| IBIS file stm32mp251_253_255_257_tfbga361.ibs
[IBIS ver] 5.1
[File name] stm32mp251_253_255_257_tfbga361.ibs
[File Rev] 1.3
[Date] 09-10-2025
[Source] Data Created at STMicroelectronics
[Notes]  File originated from ELDO simulations.
[Disclaimer]  This information is for modeling purpose only and is
   not guaranted. The information is subject to change without
   notice.
[Copyright] Copyright 2025 STMicroelectronics Inc.
|   Component stm32mp251_253_255_257_tfbga361
[Component] stm32mp251_253_255_257_tfbga361
[Manufacturer] STMicroelectronics
[Package]
| variable   typ   min   max
R_pkg  0  NA  NA
L_pkg  0  NA  NA
C_pkg  0  NA  NA
[Pin]   signal_name   model_name
A1  VSS  gnd
A2  DSI_D3N  DPHY_IBIS
A3  DSI_D2N  DPHY_IBIS
A4  DSI_CKP  DPHY_IBIS
A5  DSI_D1N  DPHY_IBIS
A6  DSI_D0N  DPHY_IBIS
A7  VDDDSI  nc
A8  PB10  io8_tt
A9  PB0  io8_tt
A10  PB5  io8_tt_i3c
A11  PD8  io8_tt
A12  PD1  io8_tt
A13  PE0  io8_tt
A14  PE6  io8_tt
A15  PE11  io8_tt
A16  PD12  io8_tt
A17  DDR_DQ11  mal4drv27_PAD
A18  DDR_DQ9  mal4drv27_PAD
A19  VSS  gnd
B1  VDDCSI  nc
B2  DSI_D3P  DPHY_IBIS
B3  DSI_D2P  DPHY_IBIS
B4  DSI_CKN  DPHY_IBIS
B5  DSI_D1P  DPHY_IBIS
B6  DSI_D0P  DPHY_IBIS
B7  VDDA18DSI  power
B8  PB7  io8_tt
B9  PB6  io8_tt
B10  PB4  io8_tt_i3c
B11  PD0  io8_tt
B12  PD15  io8_tt_i3c
B13  PE1  io8_tt
B14  PE7  io8_tt
B15  PE9  io8_tt
B16  PB12  io8_tt
B17  DDR_DQ10  mal4drv27_PAD
B18  DDR_DQS1N  mal4drv27_PAD
B19  DDR_DQS1P  mal4drv27_PAD
C1  CSI_CKP  DPHY_IBIS_L1
C2  CSI_CKN  DPHY_IBIS_L1
C3  CSI_REXT  nc
C4  PI7  io8_tt
C5  PI6  io8_tt
C6  PG15  io8_tt
C7  DSI_REXT  nc
C8  PB1  io8_tt
C9  PB2  io8_tt
C10  PD3  io8_tt
C11  PD10  io8_tt_i3c
C12  PI10  io8_tt
C13  PE2  io8_tt
C14  PE8  io8_tt
C15  PB13  io8_tt
C16  PI11  io8_tt
C17  DDR_DQ8  mal4drv27_PAD
C18  DDR_DQ15  mal4drv27_PAD
C19  DDR_DQM1  mal4drv27_PAD
D1  CSI_D1P  DPHY_IBIS_L1
D2  CSI_D1N  DPHY_IBIS_L1
D3  VDDA18CSI  power
D4  PG8  io8_tt
D5  PI5  io8_tt
D6  PI0  io8_tt
D7  PB11  io8_tt
D8  PB8  io8_tt
D9  PD2  io8_tt
D10  PD11  io8_tt_i3c
D11  PD5  io8_tt
D12  PD14  io8_tt_i3c
D13  PE4  io8_tt
D14  PE3  io8_tt
D15  PE12  io8_tt
D16  PD13  io8_tt
D17  DDR_DQ14  mal4drv27_PAD
D18  DDR_DQ13  mal4drv27_PAD
D19  DDR_DQ12  mal4drv27_PAD
E1  CSI_D0N  DPHY_IBIS_L1
E2  CSI_D0P  DPHY_IBIS_L1
E3  PG14  io8_tt
E4  PG9  io8_tt
E5  PG10  io8_tt
E6  PG11  io8_tt
E7  PB9  io8_tt
E8  PB3  io8_tt
E9  PD9  io8_tt
E10  PD4  io8_tt
E11  PD7  io8_tt
E12  PD6  io8_tt
E13  PE5  io8_tt
E14  PE10  io8_tt
E15  PE13  io8_tt
E16  PB14  io8_tt
E17  DDR_RESETN  nc
E18  DDR_A9  mal4drv20_PAD
E19  DDR_A20  mal4drv20_PAD
F1  LVDS1_D0P  nc
F2  LVDS1_D0N  nc
F3  VDDLVDS  nc
F4  PI1  io8_tt_i3c
F5  PF14  io8_tt
F6  PG7  io8_tt
F7  VDDA18PLL3  nc
F8  VDDA18PLL2  nc
F9  VDDIO4  power
F10  VDDIO4  power
F11  VDDIO3  power
F12  VDDIO3  power
F13  VDDIO2  power
F14  VDDIO1  power
F15  PE14  io8_tt
F16  PE15  io8_tt
F17  DDR_A0  mal4drv20_PAD
F18  DDR_A11  mal4drv20_PAD
F19  DDR_A21  mal4drv20_PAD
G1  LVDS1_D1P  nc
G2  LVDS1_D1N  nc
G3  VDDA18LVDS  power
G4  PG12  io8_tt
G5  PF15  io8_tt
G6  PF13  io8_tt
G7  VSS  gnd
G8  VDDCORE  nc
G9  VSS  gnd
G10  VDDCORE  nc
G11  VSS  gnd
G12  VDDCPU  nc
G13  VSS  gnd
G14  VDDQDDR  power
G15  VSS  gnd
G16  DDR_ZQ  nc
G17  DDR_A1  mal4drv20_PAD
G18  DDR_A10  mal4drv20_PAD
G19  DDR_A22  mal4drv20_PAD
H1  LVDS1_D2P  nc
H2  LVDS1_D2N  nc
H3  PG5  io8_tt_i3c
H4  PI3  io8_tt
H5  PG13  io8_tt_i3c
H6  PI4  io8_tt
H7  VDDCORE  nc
H8  VSS  gnd
H9  VDDCORE  nc
H10  VSS  gnd
H11  VDDCPU  nc
H12  VSS  gnd
H13  VDDCPU  nc
H14  VSS  gnd
H15  VDDA18PLL1  nc
H16  VSS  gnd
H17  DDR_A25  mal4drv20_PAD
H18  DDR_A8  mal4drv20_PAD
H19  DDR_A23  mal4drv20_PAD
J1  LVDS1_D4P  nc
J2  LVDS1_D4N  nc
J3  PG6  io8_tt_i3c
J4  PI9  io8_tt
J5  PF12  io8_tt
J6  PI2  io8_tt
J7  VSS  gnd
J8  VDDCORE  nc
J9  VSS  gnd
J10  VDDCORE  nc
J11  VSS  gnd
J12  VDDCPU  nc
J13  VSS  gnd
J14  VDDQDDR  power
J15  VSS  gnd
J16  VDDA18DDR  nc
J17  DDR_A2  mal4drv20_PAD
J18  DDR_A13  mal4drv20_PAD
J19  DDR_A3  mal4drv20_PAD
K1  LVDS1_D3P  nc
K2  LVDS1_D3N  nc
K3  PZ8  io8_tt
K4  PZ6  io8_tt
K5  PC13  io8_tt
K6  V08CAP  nc
K7  VDDCORE  nc
K8  VSS  gnd
K9  VDDCORE  nc
K10  VSS  gnd
K11  VDDGPU  nc
K12  VSS  gnd
K13  VDDCPU  nc
K14  VSS  gnd
K15  VDDQDDR  power
K16  VSS  gnd
K17  DDR_VREF  nc
K18  DDR_A14  mal4drv20_PAD
K19  DDR_A26  mal4drv20_PAD
L1  PZ9  io8_tt_i3c
L2  PZ7  io8_tt
L3  PZ2  io8_tt_i3c
L4  PZ4  io8_tt_i3c
L5  PZ0  io8_tt_i3c
L6  VBAT  power
L7  VSS  gnd
L8  VDD  power
L9  VSS  gnd
L10  VDD  power
L11  VSS  gnd
L12  VDDGPU  nc
L13  VSS  gnd
L14  VDDQDDR  power
L15  VSS  gnd
L16  VDDQDDR  power
L17  DDR_A5  mal4drv20_PAD
L18  DDR_A15  mal4drv20_PAD
L19  DDR_A27  mal4drv20_PAD
M1  OSC32_OUT  isudq_tt
M2  OSC32_IN  isudq_tt
M3  PZ1  io8_tt_i3c
M4  PZ5  io8_tt
M5  PZ3  io8_tt_i3c
M6  VDDA18AON  power
M7  VSSAON  gnd
M8  VSS  gnd
M9  VDD  power
M10  VSS  gnd
M11  VDDGPU  nc
M12  VSS  gnd
M13  VDDGPU  nc
M14  VSS  gnd
M15  VDDQDDR  power
M16  VSS  gnd
M17  DDR_A4  mal4drv20_PAD
M18  DDR_A16  mal4drv20_PAD
M19  DDR_A28  mal4drv20_PAD
N1  NRST  nc
N2  PWR_CPUON  io8_tt
N3  BOOT0  isudq_tt
N4  BOOT1  isudq_tt
N5  PI8  io8_tt
N6  VDDA18ADC  power
N7  VSSA  nc
N8  VDD  power
N9  VSS  gnd
N10  VDD  power
N11  VSS  gnd
N12  VDDGPU  nc
N13  VSS  gnd
N14  VDDQDDR  power
N15  VSS  gnd
N16  VDDQDDR  power
N17  DDR_A6  mal4drv20_PAD
N18  DDR_A17  mal4drv20_PAD
N19  DDR_A29  mal4drv20_PAD
P1  PDR_ON  nc
P2  NRSTC1MS  io8_tt
P3  PWR_ON  io8_tt
P4  BOOT3  isudq_tt
P5  PA0  io8_tt
P6  PF10  io8_tt
P7  PF5  io8_tt
P8  PA14  io8_tt
P9  PA13  io8_tt
P10  PC0  io8_tt
P11  PA6  io8_tt
P12  PA7  io8_tt
P13  PH2  io8_tt_i3c
P14  PA1  io8_tt_i3c
P15  VDDPCIECLK  nc
P16  UCPD1_CC1  nc
P17  DDR_A7  mal4drv20_PAD
P18  DDR_A18  mal4drv20_PAD
P19  DDR_A30  mal4drv20_PAD
R1  OSC_IN  isudq_tt
R2  OSC_OUT  isudq_tt
R3  BOOT2  isudq_tt
R4  PF11  io8_tt
R5  PF6  io8_tt
R6  PF7  io8_tt
R7  PC5  io8_tt_i3c
R8  PA11  io8_tt
R9  PA12  io8_tt_i3c
R10  PF0  io8_tt_i3c
R11  PF2  io8_tt_i3c
R12  PH6  io8_tt_i3c
R13  PH4  io8_tt
R14  PH5  io8_tt
R15  VDDCOMBOPHYTX  nc
R16  VDD33USB  power
R17  VDDA18USB  power
R18  DDR_A12  mal4drv20_PAD
R19  DDR_A31  mal4drv20_PAD
T1  VREFN  nc
T2  VREFP  nc
T3  PG1  io8_tt_i3c
T4  PG2  io8_tt_i3c
T5  PF8  io8_tt
T6  PC4  io8_tt
T7  PC6  io8_tt_i3c
T8  PH9  io8_tt
T9  PF3  io8_tt
T10  PA2  io8_tt_i3c
T11  PA5  io8_tt
T12  PH3  io8_tt_i3c
T13  PA4  io8_tt
T14  COMBOPHY_REXT  nc
T15  VDDA18COMBOPHY  power
T16  USB3DR_TXRTUNE  nc
T17  DDR_DQM0  mal4drv27_PAD
T18  DDR_DQ5  mal4drv27_PAD
T19  DDR_DQ4  mal4drv27_PAD
U1  JTDO_TRACESWO  io8_tt
U2  NJTRST  io8_tt
U3  PG3  io8_tt
U4  PF9  io8_tt
U5  PC11  io8_tt
U6  PC7  io8_tt
U7  PC10  io8_tt
U8  PF1  io8_tt
U9  PA15  io8_tt_i3c
U10  PH7  io8_tt_i3c
U11  PH8  io8_tt
U12  PA3  io8_tt_i3c
U13  PA8  io8_tt_i3c
U14  VDDCOMBOPHY  nc
U15  UCPD1_CC2  nc
U16  USBH_HS_TXRTUNE  nc
U17  DDR_DQ3  mal4drv27_PAD
U18  DDR_DQ7  mal4drv27_PAD
U19  DDR_DQ6  mal4drv27_PAD
V1  JTCK_SWCLK  io8_tt
V2  JTMS_SWDIO  io8_tt
V3  PG4  io8_tt
V4  PC12  io8_tt_i3c
V5  PC3  io8_tt
V6  PC8  io8_tt
V7  PH12  io8_tt
V8  PC2  io8_tt
V9  PC1  io8_tt_i3c
V10  PA9  io8_tt
V11  COMBOPHY_TX1P  synopsys_usb3_tx
V12  COMBOPHY_RX1P  synopsys_usb3_rx
V13  PCIE_CLKINP  nc
V14  ANA0  nc
V15  USBH_HS_DM  USB2_HS_IBIS
V16  USB3DR_DM  USB2_HS_IBIS
V17  DDR_DQ2  mal4drv27_PAD
V18  DDR_DQS0N  mal4drv27_PAD
V19  DDR_DQS0P  mal4drv27_PAD
W1  VSS  gnd
W2  JTDI  io8_tt
W3  PB15  io8_tt
W4  PG0  io8_tt_i3c
W5  PF4  io8_tt
W6  PC9  io8_tt
W7  PH13  io8_tt
W8  PH11  io8_tt
W9  PH10  io8_tt
W10  PA10  io8_tt
W11  COMBOPHY_TX1N  synopsys_usb3_tx
W12  COMBOPHY_RX1N  synopsys_usb3_rx
W13  PCIE_CLKINN  nc
W14  ANA1  nc
W15  USBH_HS_DP  USB2_HS_IBIS
W16  USB3DR_DP  USB2_HS_IBIS
W17  DDR_DQ1  mal4drv27_PAD
W18  DDR_DQ0  mal4drv27_PAD
W19  VSS  gnd
[Package Model]   505-fcbga-16x16-361-250304
[Pin Mapping]   pulldown_ref   pullup_ref   | Comment
A1  gnd  nc
A2  gnd  VDDA18DSI
A3  gnd  VDDA18DSI
A4  gnd  VDDA18DSI
A5  gnd  VDDA18DSI
A6  gnd  VDDA18DSI
A7  nc  nc
A8  gnd  vddio4
A9  gnd  vddio4
A10  gnd  vddio4
A11  gnd  vddio3
A12  gnd  vddio3
A13  gnd  vddio1
A14  gnd  vddio2
A15  gnd  vddio2
A16  gnd  vdd
A17  gnd  vddqddr
A18  gnd  vddqddr
A19  gnd  nc
B1  nc  nc
B2  nc  nc
B3  gnd  VDDA18DSI
B4  gnd  VDDA18DSI
B5  gnd  VDDA18DSI
B6  gnd  VDDA18DSI
B7  nc  VDDA18DSI
B8  gnd  vddio4
B9  gnd  vddio4
B10  gnd  vddio4
B11  gnd  vddio3
B12  gnd  vdd
B13  gnd  vddio1
B14  gnd  vddio2
B15  gnd  vddio2
B16  gnd  vdd
B17  gnd  vddqddr
B18  gnd  vddqddr
B19  gnd  vddqddr
C1  gnd  VDDA18CSI
C2  gnd  VDDA18CSI
C3  nc  nc
C4  gnd  vdd
C5  gnd  vdd
C6  gnd  vdd
C7  nc  nc
C8  gnd  vddio4
C9  gnd  vddio4
C10  gnd  vddio3
C11  gnd  vddio3
C12  gnd  vdd
C13  gnd  vddio1
C14  gnd  vddio2
C15  gnd  vdd
C16  gnd  vdd
C17  gnd  vddqddr
C18  gnd  vddqddr
C19  gnd  vddqddr
D1  gnd  VDDA18CSI
D2  gnd  VDDA18CSI
D3  nc  VDDA18CSI
D4  gnd  vdd
D5  gnd  vdd
D6  gnd  vdd
D7  gnd  vddio4
D8  gnd  vddio4
D9  gnd  vddio3
D10  gnd  vddio3
D11  gnd  vddio3
D12  gnd  vdd
D13  gnd  vddio1
D14  gnd  vddio1
D15  gnd  vddio2
D16  gnd  vdd
D17  gnd  vddqddr
D18  gnd  vddqddr
D19  gnd  vddqddr
E1  gnd  VDDA18CSI
E2  gnd  VDDA18CSI
E3  gnd  vdd
E4  gnd  vdd
E5  gnd  vdd
E6  gnd  vdd
E7  gnd  vddio4
E8  gnd  vddio4
E9  gnd  vddio3
E10  gnd  vddio3
E11  gnd  vddio3
E12  gnd  vddio3
E13  gnd  vddio1
E14  gnd  vddio2
E15  gnd  vddio2
E16  gnd  vdd
E17  nc  nc
E18  gnd  vddqddr
E19  gnd  vddqddr
F1  nc  nc
F2  nc  nc
F3  nc  nc
F4  gnd  vdd
F5  gnd  vdd
F6  gnd  vdd
F7  nc  nc
F8  nc  nc
F9  nc  vddio4
F10  nc  vddio4
F11  nc  vddio3
F12  nc  vddio3
F13  nc  vddio2
F14  nc  vddio1
F15  gnd  vddio2
F16  gnd  vddio2
F17  gnd  vddqddr
F18  gnd  vddqddr
F19  gnd  vddqddr
G1  nc  nc
G2  nc  nc
G3  nc  vdda18lvds
G4  gnd  vdd
G5  gnd  vdd
G6  gnd  vdd
G7  gnd  nc
G8  nc  nc
G9  gnd  nc
G10  nc  nc
G11  gnd  nc
G12  nc  nc
G13  gnd  nc
G14  nc  vddqddr
G15  gnd  nc
G16  nc  nc
G17  gnd  vddqddr
G18  gnd  vddqddr
G19  gnd  vddqddr
H1  nc  nc
H2  nc  nc
H3  gnd  vdd
H4  gnd  vdd
H5  gnd  vdd
H6  gnd  vdd
H7  nc  nc
H8  gnd  nc
H9  nc  nc
H10  gnd  nc
H11  nc  nc
H12  gnd  nc
H13  nc  nc
H14  gnd  nc
H15  nc  nc
H16  gnd  nc
H17  gnd  vddqddr
H18  gnd  vddqddr
H19  gnd  vddqddr
J1  nc  nc
J2  nc  nc
J3  gnd  vdd
J4  gnd  vdd
J5  gnd  vdd
J6  gnd  vdd
J7  gnd  nc
J8  nc  nc
J9  gnd  nc
J10  nc  nc
J11  gnd  nc
J12  nc  nc
J13  gnd  nc
J14  nc  vddqddr
J15  gnd  nc
J16  nc  nc
J17  gnd  vddqddr
J18  gnd  vddqddr
J19  gnd  vddqddr
K1  nc  nc
K2  nc  nc
K3  gnd  vdd
K4  gnd  vdd  | Depending on IO usage
| K4  gnd  vsw  | Depending on IO usage
K5  gnd  vdd  | Depending on IO usage
| K5  gnd  vsw  | Depending on IO usage
K6  nc  nc
K7  nc  nc
K8  gnd  nc
K9  nc  nc
K10  gnd  nc
K11  nc  nc
K12  gnd  nc
K13  nc  nc
K14  gnd  nc
K15  nc  vddqddr
K16  gnd  nc
K17  nc  nc
K18  gnd  vddqddr
K19  gnd  vddqddr
L1  gnd  vdd
L2  gnd  vdd
L3  gnd  vdd  | Depending on IO usage
| L3  gnd  vsw  | Depending on IO usage
L4  gnd  vdd  | Depending on IO usage
| L4  gnd  vsw  | Depending on IO usage
L5  gnd  vdd  | Depending on IO usage
| L5  gnd  vsw  | Depending on IO usage
L6  nc  vsw
L7  gnd  nc
L8  nc  vdd
L9  gnd  nc
L10  nc  vdd
L11  gnd  nc
L12  nc  nc
L13  gnd  nc
L14  nc  vddqddr
L15  gnd  nc
L16  nc  vddqddr
L17  gnd  vddqddr
L18  gnd  vddqddr
L19  gnd  vddqddr
M1  gnd  vdd  | Depending on IO usage
| M1  gnd  vsw  | Depending on IO usage
M2  gnd  vdd  | Depending on IO usage
| M2  gnd  vsw  | Depending on IO usage
M3  gnd  vdd  | Depending on IO usage
| M3  gnd  vsw  | Depending on IO usage
M4  gnd  vdd  | Depending on IO usage
| M4  gnd  vsw  | Depending on IO usage
M5  gnd  vdd  | Depending on IO usage
| M5  gnd  vsw  | Depending on IO usage
M6  nc  vdda18aon
M7  gnd_aon  nc
M8  gnd  nc
M9  nc  vdd
M10  gnd  nc
M11  nc  nc
M12  gnd  nc
M13  nc  nc
M14  gnd  nc
M15  nc  vddqddr
M16  gnd  nc
M17  gnd  vddqddr
M18  gnd  vddqddr
M19  gnd  vddqddr
N1  nc  nc
N2  gnd  vdd
N3  gnd  vdd
N4  gnd  vdd
N5  gnd  vdd  | Depending on IO usage
| N5  gnd  vsw  | Depending on IO usage
N6  nc  vdda18adc
N7  nc  nc
N8  nc  vdd
N9  gnd  nc
N10  nc  vdd
N11  gnd  nc
N12  nc  nc
N13  gnd  nc
N14  nc  vddqddr
N15  gnd  nc
N16  nc  vddqddr
N17  gnd  vddqddr
N18  gnd  vddqddr
N19  gnd  vddqddr
P1  nc  nc
P2  gnd  vdd
P3  gnd  vdd
P4  gnd  vdd
P5  gnd  vdd
P6  gnd  vdd
P7  gnd  vdd
P8  gnd  vdd
P9  gnd  vdd
P10  gnd  vdd
P11  gnd  vdd
P12  gnd  vdd
P13  gnd  vdd
P14  gnd  vdd
P15  nc  nc
P16  nc  nc
P17  gnd  vddqddr
P18  gnd  vddqddr
P19  gnd  vddqddr
R1  gnd_aon  vdda18aon
R2  gnd_aon  vdda18aon
R3  gnd  vdd
R4  gnd  vdd
R5  gnd  vdd  | Depending on IO usage
| R5  gnd  vsw  | Depending on IO usage
R6  gnd  vdd  | Depending on IO usage
| R6  gnd  vsw  | Depending on IO usage
R7  gnd  vdd  | Depending on IO usage
| R7  gnd  vsw  | Depending on IO usage
R8  gnd  vdd
R9  gnd  vdd
R10  gnd  vdd
R11  gnd  vdd
R12  gnd  vdd
R13  gnd  vdd
R14  gnd  vdd
R15  nc  nc
R16  nc  VDD33USB
R17  nc  vdda18usb
R18  gnd  vddqddr
R19  gnd  vddqddr
T1  nc  nc
T2  nc  nc
T3  gnd  vdd  | Depending on IO usage
| T3  gnd  vsw  | Depending on IO usage
T4  gnd  vdd
T5  gnd  vdd
T6  gnd  vdd  | Depending on IO usage
| T6  gnd  vsw  | Depending on IO usage
T7  gnd  vdd
T8  gnd  vdd
T9  gnd  vdd
T10  gnd  vdd
T11  gnd  vdd
T12  gnd  vdd
T13  gnd  vdd
T14  nc  nc
T15  nc  vdda18combophy
T16  nc  nc
T17  gnd  vddqddr
T18  gnd  vddqddr
T19  gnd  vddqddr
U1  gnd  vdd
U2  gnd  vdd
U3  gnd  vdd  | Depending on IO usage
| U3  gnd  vsw  | Depending on IO usage
U4  gnd  vdd
U5  gnd  vdd
U6  gnd  vdd
U7  gnd  vdd
U8  gnd  vdd
U9  gnd  vdd
U10  gnd  vdd
U11  gnd  vdd
U12  gnd  vdd
U13  gnd  vdd
U14  nc  nc
U15  nc  nc
U16  nc  nc
U17  gnd  vddqddr
U18  gnd  vddqddr
U19  gnd  vddqddr
V1  gnd  vdd
V2  gnd  vdd
V3  gnd  vdd
V4  gnd  vdd
V5  gnd  vdd  | Depending on IO usage
| V5  gnd  vsw  | Depending on IO usage
V6  gnd  vdd
V7  gnd  vdd
V8  gnd  vdd
V9  gnd  vdd
V10  gnd  vdd
V11  gnd  vdda18combophy
V12  gnd  vdda18combophy
V13  nc  nc
V14  nc  nc
V15  gnd  VDD33USB
V16  gnd  VDD33USB
V17  gnd  vddqddr
V18  gnd  vddqddr
V19  gnd  vddqddr
W1  gnd  nc
W2  gnd  vdd
W3  gnd  vdd
W4  gnd  vdd
W5  gnd  vdd
W6  gnd  vdd
W7  gnd  vdd
W8  gnd  vdd
W9  gnd  vdd
W10  gnd  vdd
W11  gnd  vdda18combophy
W12  gnd  vdda18combophy
W13  nc  nc
W14  nc  nc
W15  gnd  VDD33USB
W16  gnd  VDD33USB
W17  gnd  vddqddr
W18  gnd  vddqddr
W19  gnd  nc
[Diff Pin]  inv_pin  vdiff  tdelay_typ  tdelay_min  tdelay_max
M17  L17  0.320V 0ns  NA  NA  |CK
V19  V18  0.320V 0ns  NA  NA  |DQS0
B19  B18  0.320V 0ns  NA  NA  |DQS1
V12  W12  NA  NA  NA  NA
V11  W11  NA  NA  NA  NA
C1  C2  NA  NA  NA  NA
E2  E1  NA  NA  NA  NA
D1  D2  NA  NA  NA  NA
A4  B4  NA  NA  NA  NA   |DSI CKP CKN
B6  A6  400.000mV   0ns   NA   NA   |D0P D0N
B5  A5  400.000mV   0ns   NA   NA   |D1P D1N
B3  A3  400.000mV   0ns   NA   NA   |D2P D2N
B2  A2  400.000mV   0ns   NA   NA   |D3P D3N
F1  F2  NA  NA  NA  NA
G1  G2  NA  NA  NA  NA
H1  H2  NA  NA  NA  NA
K1  K2  NA  NA  NA  NA
J1  J2  NA  NA  NA  NA
V13  W13  NA  NA  NA  NA
W16  V16  NA  NA  NA  NA   |USB3DR_DP _DM
W15  V15  NA  NA  NA  NA   |USBH_HS_DP _DM
[Model Selector] DPHY_IBIS_L1
DPHY_RX_2P5G_L1   DPHY HSRX model at 2.5Gbps for lane 1
DPHY_RX_1P5G_L1   DPHY HSRX model at 1.5Gbps for lane 1
[Model Selector] DPHY_IBIS
DPHY_TX_2P5G   DPHY HSTX model at 2.5Gbps
DPHY_TX_1P5G   DPHY HSTX model at 1.5Gbps
[Model Selector] USB2_HS_IBIS
USB2_HSRX   USB2 HSRX model
USB2_HSTX_00_0_01_0011_11   TuningBits_AMP_PULSE_RISE_REF_XV=00_0_01_0011_11
USB2_HSTX_00_0_10_0101_11   TuningBits_AMP_PULSE_RISE_REF_XV=00_0_10_0101_11
USB2_HSTX_00_0_11_0111_11   TuningBits_AMP_PULSE_RISE_REF_XV=00_0_11_0111_11
USB2_HSTX_00_1_01_0011_11   TuningBits_AMP_PULSE_RISE_REF_XV=00_1_01_0011_11
USB2_HSTX_00_1_10_0101_11   TuningBits_AMP_PULSE_RISE_REF_XV=00_1_10_0101_11
USB2_HSTX_00_1_11_0111_11   TuningBits_AMP_PULSE_RISE_REF_XV=00_1_11_0111_11
USB2_HSTX_01_0_01_0011_11   TuningBits_AMP_PULSE_RISE_REF_XV=01_0_01_0011_11
USB2_HSTX_01_0_10_0101_11   TuningBits_AMP_PULSE_RISE_REF_XV=01_0_10_0101_11
USB2_HSTX_01_0_11_0111_11   TuningBits_AMP_PULSE_RISE_REF_XV=01_0_11_0111_11
USB2_HSTX_01_1_01_0011_11   TuningBits_AMP_PULSE_RISE_REF_XV=01_1_01_0011_11
USB2_HSTX_01_1_10_0101_11   TuningBits_AMP_PULSE_RISE_REF_XV=01_1_10_0101_11
USB2_HSTX_01_1_11_0111_11   TuningBits_AMP_PULSE_RISE_REF_XV=01_1_11_0111_11
USB2_HSTX_10_0_01_0011_11   TuningBits_AMP_PULSE_RISE_REF_XV=10_0_01_0011_11
USB2_HSTX_10_0_10_0101_11   TuningBits_AMP_PULSE_RISE_REF_XV=10_0_10_0101_11
USB2_HSTX_10_0_11_0111_11   TuningBits_AMP_PULSE_RISE_REF_XV=10_0_11_0111_11
USB2_HSTX_10_1_01_0011_11   TuningBits_AMP_PULSE_RISE_REF_XV=10_1_01_0011_11
USB2_HSTX_10_1_10_0101_11   TuningBits_AMP_PULSE_RISE_REF_XV=10_1_10_0101_11
USB2_HSTX_10_1_11_0111_11   TuningBits_AMP_PULSE_RISE_REF_XV=10_1_11_0111_11
[Model Selector] io8_tt
io8_tt_ls_3v3 "GPIO - 3V tolerant - low speed - 3.3V range"
io8_tt_ms_3v3 "GPIO - 3V tolerant - med speed - 3.3V range"
io8_tt_fs_3v3 "GPIO - 3V tolerant - fast speed - 3.3V range"
io8_tt_hs_3v3 "GPIO - 3V tolerant - high speed - 3.3V range"
io8_tt_hslv_ls_1v8 "GPIO low voltage optimization - 3V tolerant - low speed - 1.8V range"
io8_tt_hslv_ms_1v8 "GPIO low voltage optimization - 3V tolerant - med speed - 1.8V range"
io8_tt_hslv_fs_1v8 "GPIO low voltage optimization - 3V tolerant - fast speed - 1.8V range"
io8_tt_hslv_hs_1v8 "GPIO low voltage optimization - 3V tolerant - high speed - 1.8V range"
[Model Selector] io8_tt_i3c
io8_tt_ls_3v3 "GPIO - 3V tolerant - low speed - 3.3V range"
io8_tt_ms_3v3 "GPIO - 3V tolerant - med speed - 3.3V range"
io8_tt_fs_3v3 "GPIO - 3V tolerant - fast speed - 3.3V range"
io8_tt_hs_3v3 "GPIO - 3V tolerant - high speed - 3.3V range"
io8_tt_hslv_ls_1v8 "GPIO low voltage optimization - 3V tolerant - low speed - 1.8V range"
io8_tt_hslv_ms_1v8 "GPIO low voltage optimization - 3V tolerant - med speed - 1.8V range"
io8_tt_hslv_fs_1v8 "GPIO low voltage optimization - 3V tolerant - fast speed - 1.8V range"
io8_tt_hslv_hs_1v8 "GPIO low voltage optimization - 3V tolerant - high speed - 1.8V range"
io8_tt_i3c_ls_3v3 "GPIO with I3C open-drain - 3V tolerant - low speed - 3.3V range"
io8_tt_i3c_ms_3v3 "GPIO with I3C open-drain - 3V tolerant - med speed - 3.3V range"
io8_tt_i3c_fs_3v3 "GPIO with I3C open-drain - 3V tolerant - fast speed - 3.3V range"
io8_tt_i3c_hs_3v3 "GPIO with I3C open-drain - 3V tolerant - high speed - 3.3V range"
io8_tt_hslv_i3c_ls_1v8 "GPIO low voltage optimization with I3C open-drain - 3V tolerant - low speed - 1.8V range"
io8_tt_hslv_i3c_ms_1v8 "GPIO low voltage optimization with I3C open-drain - 3V tolerant - med speed - 1.8V range"
io8_tt_hslv_i3c_fs_1v8 "GPIO low voltage optimization with I3C open-drain - 3V tolerant - fast speed - 1.8V range"
io8_tt_hslv_i3c_hs_1v8 "GPIO low voltage optimization with I3C open-drain - 3V tolerant - high speed - 1.8V range"
io8_tt_i3c_fmp_3v3 "GPIO with I3C fm+ open-drain - 3V tolerant - 3.3V range"
[Model Selector] isudq_tt
isudq_tt_3v3 "Input Buffer - 3V tolerant - 3.3V range"
isudq_tt_1v8 "Input Buffer - 3V tolerant - 1.8V range"
[Model Selector]   mal4drv20_PAD
mal4drv20_d3l_40   DDR3L mal4drv20 cell  Z0=40-Ohm Driver
mal4drv20_d3l_60   DDR3L mal4drv20 cell  Z0=60-Ohm Driver
mal4drv20_d3l_120   DDR3L mal4drv20 cell  Z0=120-Ohm Driver
mal4drv20_d3_20   DDR3 mal4drv20 cell  Z0=20-Ohm Driver
mal4drv20_d3_24   DDR3 mal4drv20 cell  Z0=24-Ohm Driver
mal4drv20_d3_30   DDR3 mal4drv20 cell  Z0=30-Ohm Driver
mal4drv20_d3_40   DDR3 mal4drv20 cell  Z0=40-Ohm Driver
mal4drv20_d3_60   DDR3 mal4drv20 cell  Z0=60-Ohm Driver
mal4drv20_d4_20   DDR4 mal4drv20 cell  Z0=20-Ohm Driver
mal4drv20_d4_24   DDR4 mal4drv20 cell  Z0=24-Ohm Driver
mal4drv20_d4_30   DDR4 mal4drv20 cell  Z0=30-Ohm Driver
mal4drv20_d4_40   DDR4 mal4drv20 cell  Z0=40-Ohm Driver
mal4drv20_d4_60   DDR4 mal4drv20 cell  Z0=60-Ohm Driver
mal4drv20_dl4_20   LPDDR4 mal4drv20 cell  Z0=20-Ohm Driver
mal4drv20_dl4_24   LPDDR4 mal4drv20 cell  Z0=24-Ohm Driver
mal4drv20_dl4_30   LPDDR4 mal4drv20 cell  Z0=30-Ohm Driver
mal4drv20_dl4_40   LPDDR4 mal4drv20 cell  Z0=40-Ohm Driver
mal4drv20_dl4_60   LPDDR4 mal4drv20 cell  Z0=60-Ohm Driver
[Model Selector]   mal4drv27_PAD
mal4drv27_d3l_40   DDR3L mal4drv27 cell  Z0=40-Ohm Driver
mal4drv27_d3l_48   DDR3L mal4drv27 cell  Z0=48-Ohm Driver
mal4drv27_d3l_60   DDR3L mal4drv27 cell  Z0=60-Ohm Driver
mal4drv27_d3l_80   DDR3L mal4drv27 cell  Z0=80-Ohm Driver
mal4drv27_d3l_120   DDR3L mal4drv27 cell  Z0=120-Ohm Driver
mal4drv27_d3l_240   DDR3L mal4drv27 cell  Z0=240-Ohm Driver
mal4drv27_d3l_odt120   DDR3L mal4drv27 cell 120-Ohm ODT Receiver
mal4drv27_d3l_odt60   DDR3L mal4drv27 cell 60-Ohm ODT Receiver
mal4drv27_d3l_odtoff   DDR3L mal4drv27 cell ODT OFF Receiver
mal4drv27_d3_28   DDR3 mal4drv27 cell  Z0=28-Ohm Driver
mal4drv27_d3_34   DDR3 mal4drv27 cell  Z0=34-Ohm Driver
mal4drv27_d3_40   DDR3 mal4drv27 cell  Z0=40-Ohm Driver
mal4drv27_d3_53   DDR3 mal4drv27 cell  Z0=53-Ohm Driver
mal4drv27_d3_odt120   DDR3 mal4drv27 cell 120-Ohm ODT Receiver
mal4drv27_d3_odt60   DDR3 mal4drv27 cell 60-Ohm ODT Receiver
mal4drv27_d4_28   DDR4 mal4drv27 cell  Z0=28-Ohm Driver
mal4drv27_d4_34   DDR4 mal4drv27 cell  Z0=34-Ohm Driver
mal4drv27_d4_40   DDR4 mal4drv27 cell  Z0=40-Ohm Driver
mal4drv27_d4_53   DDR4 mal4drv27 cell  Z0=53-Ohm Driver
mal4drv27_d4_odt120   DDR4 mal4drv27 cell 120-Ohm ODT Receiver
mal4drv27_d4_odt240   DDR4 mal4drv27 cell 240-Ohm ODT Receiver
mal4drv27_d4_odt48   DDR4 mal4drv27 cell 48-Ohm ODT Receiver
mal4drv27_d4_odt60   DDR4 mal4drv27 cell 60-Ohm ODT Receiver
mal4drv27_d4_odt80   DDR4 mal4drv27 cell 80-Ohm ODT Receiver
mal4drv27_dl4_28   LPDDR4 mal4drv27 cell  Z0=28-Ohm Driver
mal4drv27_dl4_34   LPDDR4 mal4drv27 cell  Z0=34-Ohm Driver
mal4drv27_dl4_40   LPDDR4 mal4drv27 cell  Z0=40-Ohm Driver
mal4drv27_dl4_53   LPDDR4 mal4drv27 cell  Z0=53-Ohm Driver
mal4drv27_dl4_odt48   LPDDR4 mal4drv27 cell 48-Ohm ODT Receiver
mal4drv27_dl4_odt60   LPDDR4 mal4drv27 cell 60-Ohm ODT Receiver
[Define Package Model]  505-fcbga-16x16-361-250304
[Manufacturer]  unknown
[OEM]  unknown
[Description]  unknown
[Number Of Pins]  296
[Pin Numbers]
| Pin Name Terminal   Net Name   Starting Node   Ending Node
V14 | ANA0
W14 | ANA1
N3 | BOOT0
N4 | BOOT1
R3 | BOOT2
P4 | BOOT3
T14 | COMBOPHY_REXT
W12 | COMBOPHY_RX1N
V12 | COMBOPHY_RX1P
W11 | COMBOPHY_TX1N
V11 | COMBOPHY_TX1P
C2 | CSI_CKN
C1 | CSI_CKP
E1 | CSI_D0N
E2 | CSI_D0P
D2 | CSI_D1N
D1 | CSI_D1P
C3 | CSI_REXT
F17 | DDR_A0
G17 | DDR_A1
J17 | DDR_A2
J19 | DDR_A3
M17 | DDR_A4
L17 | DDR_A5
N17 | DDR_A6
P17 | DDR_A7
H18 | DDR_A8
E18 | DDR_A9
G18 | DDR_A10
F18 | DDR_A11
R18 | DDR_A12
J18 | DDR_A13
K18 | DDR_A14
L18 | DDR_A15
M18 | DDR_A16
N18 | DDR_A17
P18 | DDR_A18
E19 | DDR_A20
F19 | DDR_A21
G19 | DDR_A22
H19 | DDR_A23
H17 | DDR_A25
K19 | DDR_A26
L19 | DDR_A27
M19 | DDR_A28
N19 | DDR_A29
P19 | DDR_A30
R19 | DDR_A31
W18 | DDR_DQ0
W17 | DDR_DQ1
V17 | DDR_DQ2
U17 | DDR_DQ3
T19 | DDR_DQ4
T18 | DDR_DQ5
U19 | DDR_DQ6
U18 | DDR_DQ7
C17 | DDR_DQ8
A18 | DDR_DQ9
B17 | DDR_DQ10
A17 | DDR_DQ11
D19 | DDR_DQ12
D18 | DDR_DQ13
D17 | DDR_DQ14
C18 | DDR_DQ15
T17 | DDR_DQM0
C19 | DDR_DQM1
V18 | DDR_DQS0N
V19 | DDR_DQS0P
B18 | DDR_DQS1N
B19 | DDR_DQS1P
E17 | DDR_RESETN
K17 | DDR_VREF
G16 | DDR_ZQ
B4 | DSI_CKN
A4 | DSI_CKP
A6 | DSI_D0N
B6 | DSI_D0P
A5 | DSI_D1N
B5 | DSI_D1P
A3 | DSI_D2N
B3 | DSI_D2P
A2 | DSI_D3N
B2 | DSI_D3P
C7 | DSI_REXT
V1 | JTCK_SWCLK
W2 | JTDI
U1 | JTDO_TRACESWO
V2 | JTMS_SWDIO
F2 | LVDS1_D0N
F1 | LVDS1_D0P
G2 | LVDS1_D1N
G1 | LVDS1_D1P
H2 | LVDS1_D2N
H1 | LVDS1_D2P
K2 | LVDS1_D3N
K1 | LVDS1_D3P
J2 | LVDS1_D4N
J1 | LVDS1_D4P
U2 | NJTRST
N1 | NRST
P2 | NRSTC1MS
M2 | OSC32_IN
M1 | OSC32_OUT
R1 | OSC_IN
R2 | OSC_OUT
T16 | USB3DR_TXRTUNE
P5 | PA0
P14 | PA1
T10 | PA2
U12 | PA3
T13 | PA4
T11 | PA5
P11 | PA6
P12 | PA7
U13 | PA8
V10 | PA9
W10 | PA10
R8 | PA11
R9 | PA12
P9 | PA13
P8 | PA14
U9 | PA15
A9 | PB0
C8 | PB1
C9 | PB2
E8 | PB3
B10 | PB4
A10 | PB5
B9 | PB6
B8 | PB7
D8 | PB8
E7 | PB9
A8 | PB10
D7 | PB11
B16 | PB12
C15 | PB13
E16 | PB14
W3 | PB15
P10 | PC0
V9 | PC1
V8 | PC2
V5 | PC3
T6 | PC4
R7 | PC5
T7 | PC6
U6 | PC7
V6 | PC8
W6 | PC9
U7 | PC10
U5 | PC11
V4 | PC12
K5 | PC13
W13 | PCIE_CLKINN
V13 | PCIE_CLKINP
B11 | PD0
A12 | PD1
D9 | PD2
C10 | PD3
E10 | PD4
D11 | PD5
E12 | PD6
E11 | PD7
A11 | PD8
E9 | PD9
C11 | PD10
D10 | PD11
A16 | PD12
D16 | PD13
D12 | PD14
B12 | PD15
P1 | PDR_ON
A13 | PE0
B13 | PE1
C13 | PE2
D14 | PE3
D13 | PE4
E13 | PE5
A14 | PE6
B14 | PE7
C14 | PE8
B15 | PE9
E14 | PE10
A15 | PE11
D15 | PE12
E15 | PE13
F15 | PE14
F16 | PE15
R10 | PF0
U8 | PF1
R11 | PF2
T9 | PF3
W5 | PF4
P7 | PF5
R5 | PF6
R6 | PF7
T5 | PF8
U4 | PF9
P6 | PF10
R4 | PF11
J5 | PF12
G6 | PF13
F5 | PF14
G5 | PF15
W4 | PG0
T3 | PG1
T4 | PG2
U3 | PG3
V3 | PG4
H3 | PG5
J3 | PG6
F6 | PG7
D4 | PG8
E4 | PG9
E5 | PG10
E6 | PG11
G4 | PG12
H5 | PG13
E3 | PG14
C6 | PG15
P13 | PH2
T12 | PH3
R13 | PH4
R14 | PH5
R12 | PH6
U10 | PH7
U11 | PH8
T8 | PH9
W9 | PH10
W8 | PH11
V7 | PH12
W7 | PH13
D6 | PI0
F4 | PI1
J6 | PI2
H4 | PI3
H6 | PI4
D5 | PI5
C5 | PI6
C4 | PI7
N5 | PI8
J4 | PI9
C12 | PI10
C16 | PI11
N2 | PWR_CPUON
P3 | PWR_ON
L5 | PZ0
M3 | PZ1
L3 | PZ2
M5 | PZ3
L4 | PZ4
M4 | PZ5
K4 | PZ6
L2 | PZ7
K3 | PZ8
L1 | PZ9
P16 | UCPD1_CC1
U15 | UCPD1_CC2
V16 | USB3DR_DM
W16 | USB3DR_DP
V15 | USBH_HS_DM
W15 | USBH_HS_DP
U16 | USBH_HS_TXRTUNE
K6 | V08CAP
L6 | VBAT
R16 | VDD33USB
L8 | VDD
N6 | VDDA18ADC
M6 | VDDA18AON
T15 | VDDA18COMBOPHY
D3 | VDDA18CSI
J16 | VDDA18DDR
B7 | VDDA18DSI
G3 | VDDA18LVDS
H15 | VDDA18PLL1
F8 | VDDA18PLL2
F7 | VDDA18PLL3
R17 | VDDA18USB
U14 | VDDCOMBOPHY
R15 | VDDCOMBOPHYTX
G8 | VDDCORE
G12 | VDDCPU
B1 | VDDCSI
A7 | VDDDSI
K11 | VDDGPU
F14 | VDDIO1
F13 | VDDIO2
F11 | VDDIO3
F9 | VDDIO4
F3 | VDDLVDS
P15 | VDDPCIECLK
G14 | VDDQDDR
T1 | VREFN
T2 | VREFP
A1 | VSS
N7 | VSSA
M7 | VSSAON
|[Merged Pins]  L8
|L10  |  VDD
|M9  |  VDD
|N8  |  VDD
|N10  |  VDD
|[Merged Pins]  G8
|G10  |  VDDCORE
|H7  |  VDDCORE
|H9  |  VDDCORE
|J8  |  VDDCORE
|J10  |  VDDCORE
|K7  |  VDDCORE
|K9  |  VDDCORE
|[Merged Pins]  G12
|H11  |  VDDCPU
|H13  |  VDDCPU
|J12  |  VDDCPU
|K13  |  VDDCPU
|[Merged Pins]  K11
|L12  |  VDDGPU
|M11  |  VDDGPU
|M13  |  VDDGPU
|N12  |  VDDGPU
|[Merged Pins]  F11
|F12  |  VDDIO3
|[Merged Pins]  F9
|F10  |  VDDIO4
|[Merged Pins]  G14
|J14  |  VDDQDDR
|K15  |  VDDQDDR
|L14  |  VDDQDDR
|L16  |  VDDQDDR
|M15  |  VDDQDDR
|N14  |  VDDQDDR
|N16  |  VDDQDDR
|[Merged Pins]  A1
|A19  |  VSS
|G7  |  VSS
|G9  |  VSS
|G11  |  VSS
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[Model Data]
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[End Model Data]
[End Package Model]
|End [Component]
| Models and submodels in the file (92): synopsys_usb3_tx (Output), synopsys_usb3_rx (Input), USB2_HSRX (Input), USB2_HSTX_00_0_01_0011_11 (Output), USB2_HSTX_00_0_10_0101_11 (Output), USB2_HSTX_00_0_11_0111_11 (Output), USB2_HSTX_00_1_01_0011_11 (Output), USB2_HSTX_00_1_10_0101_11 (Output), USB2_HSTX_00_1_11_0111_11 (Output), USB2_HSTX_01_0_01_0011_11 (Output), USB2_HSTX_01_0_10_0101_11 (Output), USB2_HSTX_01_0_11_0111_11 (Output), USB2_HSTX_01_1_01_0011_11 (Output), USB2_HSTX_01_1_10_0101_11 (Output), USB2_HSTX_01_1_11_0111_11 (Output), USB2_HSTX_10_0_01_0011_11 (Output), USB2_HSTX_10_0_10_0101_11 (Output), USB2_HSTX_10_0_11_0111_11 (Output), USB2_HSTX_10_1_01_0011_11 (Output), USB2_HSTX_10_1_10_0101_11 (Output), USB2_HSTX_10_1_11_0111_11 (Output), DPHY_TX_2P5G (Output), DPHY_TX_1P5G (Output), DPHY_RX_1P5G_L1 (Input), DPHY_RX_2P5G_L1 (Input), io8_tt_fs_3v3 (I/O), io8_tt_hs_3v3 (I/O), io8_tt_hslv_fs_1v8 (I/O), io8_tt_hslv_hs_1v8 (I/O), io8_tt_hslv_i3c_fs_1v8 (I/O_open_drain), io8_tt_hslv_i3c_hs_1v8 (I/O_open_drain), io8_tt_hslv_i3c_ls_1v8 (I/O_open_drain), io8_tt_hslv_i3c_ms_1v8 (I/O_open_drain), io8_tt_hslv_ls_1v8 (I/O), io8_tt_hslv_ms_1v8 (I/O), io8_tt_i3c_fmp_3v3 (I/O_open_drain), io8_tt_i3c_fs_3v3 (I/O_open_drain), io8_tt_i3c_hs_3v3 (I/O_open_drain), io8_tt_i3c_ls_3v3 (I/O_open_drain), io8_tt_i3c_ms_3v3 (I/O_open_drain), io8_tt_ls_3v3 (I/O), io8_tt_ms_3v3 (I/O), isudq_tt_1v8 (Input), isudq_tt_3v3 (Input), mal4drv20_d3_20 (I/O), mal4drv20_d3_24 (I/O), mal4drv20_d3_30 (I/O), mal4drv20_d3_40 (I/O), mal4drv20_d3_60 (I/O), mal4drv20_d4_20 (I/O), mal4drv20_d4_24 (I/O), mal4drv20_d4_30 (I/O), mal4drv20_d4_40 (I/O), mal4drv20_d4_60 (I/O), mal4drv20_dl4_20 (I/O), mal4drv20_dl4_24 (I/O), mal4drv20_dl4_30 (I/O), mal4drv20_dl4_40 (I/O), mal4drv20_dl4_60 (I/O), mal4drv27_d3_28 (I/O), mal4drv27_d3_34 (I/O), mal4drv27_d3_40 (I/O), mal4drv27_d3_53 (I/O), mal4drv27_d3_odt120 (Input), mal4drv27_d3_odt60 (Input), mal4drv27_dl4_28 (I/O), mal4drv27_dl4_34 (I/O), mal4drv27_dl4_40 (I/O), mal4drv27_dl4_53 (I/O), mal4drv27_dl4_odt48 (Input), mal4drv27_dl4_odt60 (Input), mal4drv27_d4_28 (I/O), mal4drv27_d4_34 (I/O), mal4drv27_d4_40 (I/O), mal4drv27_d4_53 (I/O), mal4drv27_d4_odt120 (Input), mal4drv27_d4_odt240 (Input), mal4drv27_d4_odt48 (Input), mal4drv27_d4_odt60 (Input), mal4drv27_d4_odt80 (Input)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
